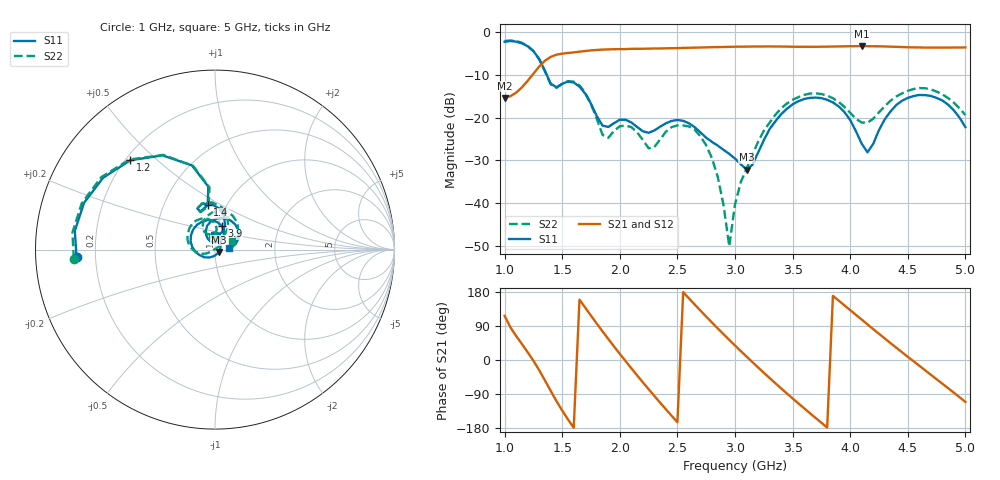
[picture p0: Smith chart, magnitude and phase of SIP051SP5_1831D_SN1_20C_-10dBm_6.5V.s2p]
# GHz  S  dB  R  50
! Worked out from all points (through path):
!   81 points, 1 GHz to 5 GHz, reference 50 ohm
!   highest |S21| = -3.27 dB at 4.1 GHz (marker M1); lowest = -15.4 dB at 1 GHz (marker M2)
!   lowest |S11| = -32.1 dB at 3.1 GHz (marker M3), VSWR 1.05, Z = 52.1 - j1.36 ohm
!   |S11| at or under -10 dB: 1.366 GHz to end of sweep
!   |S22| runs from -50.0 to -1.9 dB; largest |S21 - S12| = 0.0025
!   S11 on the Smith chart (normalised r, x): 1 GHz: 0.13, -0.03; 1.2 GHz: 0.22, +0.41; 1.4 GHz: 0.82, +0.43; 3.9 GHz: 1.04, +0.28; 5 GHz: 1.17, +0.02
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1  -2.24 -176.8  -15.41 116.4  -15.39 116.1  -2.07 -176.3
1.2  -3.28 133.5  -11.38 20.7  -11.39 20.8  -3.21 133.5
1.3  -6.26 105.3  -8.04 -26.8  -8.04 -26.8  -6.33 104.7
1.4  -12.01 99.3  -5.77 -81.4  -5.77 -81.4  -12.19 98.4
1.55  -11.54 106.3  -4.87 -156.7  -4.85 -156.7  -11.45 105.5
1.7  -14.38 74.4  -4.40 138.0  -4.41 137.9  -14.14 69.2
1.85  -21.84 79.5  -4.08 75.6  -4.07 75.6  -23.99 69.1
2.05  -20.46 94.4  -3.95 -2.8  -3.96 -3.0  -21.85 93.3
2.2  -23.17 91.8  -3.88 -58.9  -3.86 -58.9  -25.19 82.5
2.35  -22.10 104.7  -3.81 -112.6  -3.81 -112.6  -25.09 119.6
2.6  -21.30 71.3  -3.65 162.7  -3.66 162.8  -22.03 78.0
2.8  -25.64 53.9  -3.51 99.0  -3.51 98.9  -29.48 43.7
2.95  -28.44 36.5  -3.43 53.1  -3.42 53.2  -50.03 159.4
3  -29.56 24.3  -3.40 38.3  -3.40 38.3  -40.29 -158.3
3.1  -32.12 -31.8  -3.38 9.1  -3.38 9.0  -31.95 -153.6
3.4  -19.19 -173.4  -3.36 -74.8  -3.37 -74.8  -17.83 178.1
3.7  -15.29 114.6  -3.42 -153.0  -3.42 -153.0  -14.28 123.7
3.9  -17.36 73.3  -3.34 156.8  -3.34 156.7  -16.30 93.0
4.1  -26.08 63.7  -3.27 106.7  -3.26 106.5  -21.12 95.2
4.35  -18.54 115.4  -3.39 44.6  -3.40 44.6  -16.02 115.5
4.65  -14.72 61.0  -3.61 -27.0  -3.60 -27.0  -13.10 71.3
5  -22.20 6.7  -3.57 -110.5  -3.58 -110.4  -19.38 25.2
